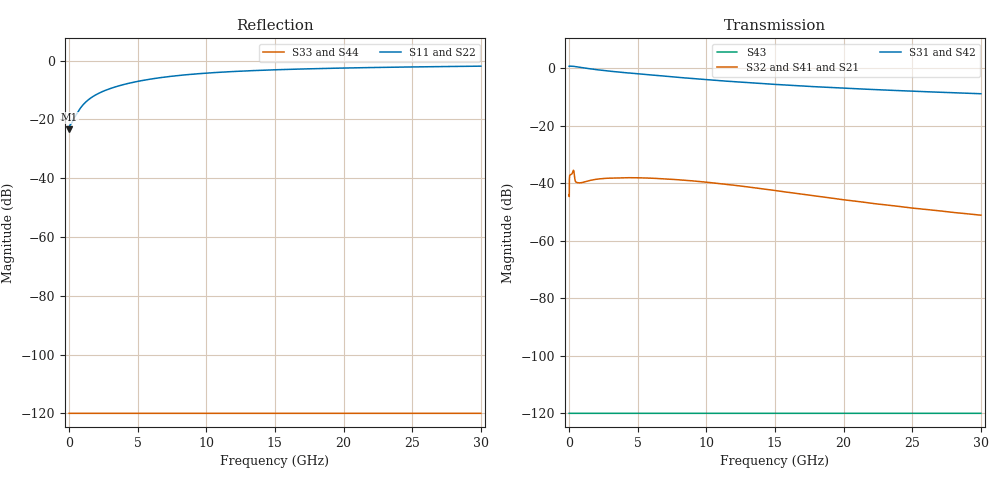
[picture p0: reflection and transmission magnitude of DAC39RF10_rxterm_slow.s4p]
! Copyright 2008, Texas Instruments Incorporated. All rights reserved.
! Generated by program util_convert_RxTerm_to_s4p on 03-29-2011 13:59:15
!  1 ----xxxxxxxxxxxxxxxxxx---- 3
!  xxxxxxxxxxxxxxxxxx
!  (Input) xxxxxxxxxxxxxxxxxx  (Output)
!  xxxxxxxxxxxxxxxxxx
!  2 ----xxxxxxxxxxxxxxxxxx---- 4
! FREQ  S11  S12  S13  S14
!  S21  S22  S23  S24
!  S31  S32  S33  S34
!  S41  S42  S43  S44
!  DB  ANG  DB  ANG  DB  ANG  DB  ANG
# HZ S DB R 50.00
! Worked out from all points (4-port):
!   3000 points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, 10 MHz to 30 GHz, reference 50 ohm
!   strongest paths, dB at 10 MHz, 7.51 GHz, 15.01 GHz, 22.51 GHz, 30 GHz:
!     S31: 0.6, -3.1, -5.7, -7.5, -8.9
!     S42: 0.6, -3.1, -5.7, -7.6, -8.9
!     S32: -44.0, -38.7, -42.6, -47.3, -51.1
!     S41: -44.0, -38.8, -42.7, -47.3, -51.1
!     S21: -44.0, -38.8, -42.7, -47.3, -51.1
!     S43: -120.0, -120.0, -120.0, -120.0, -120.0
!   lowest |S11| = -23.3 dB at 20 MHz (marker M1), VSWR 1.15, Z = 57.3 + j0.0422 ohm
!   |S11| at or under -10 dB: start of sweep to 2.716 GHz
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1e7  -22.90 -3.0  -44.03 -13.4  -120.00 0.0  -120.00 0.0
     -44.00 -13.7  -22.88 -3.0  -120.00 0.0  -120.00 0.0
     0.60 -0.2  -44.03 -13.4  -120.00 0.0  -120.00 0.0
     -44.00 -13.7  0.60 -0.2  -120.00 0.0  -120.00 0.0
2e7  -23.31 0.3  -44.69 58.3  -120.00 0.0  -120.00 0.0
     -44.87 58.3  -23.28 0.3  -120.00 0.0  -120.00 0.0
     0.57 0.0  -44.69 58.3  -120.00 0.0  -120.00 0.0
     -44.87 58.3  0.58 0.0  -120.00 0.0  -120.00 0.0
2.3e8  -20.95 -34.1  -36.63 0.3  -120.00 0.0  -120.00 0.0
       -36.66 0.6  -20.90 -34.2  -120.00 0.0  -120.00 0.0
       0.63 -2.7  -36.63 0.3  -120.00 0.0  -120.00 0.0
       -36.66 0.6  0.63 -2.7  -120.00 0.0  -120.00 0.0
6.4e8  -17.50 -74.0  -39.85 -10.8  -120.00 0.0  -120.00 0.0
       -39.85 -11.0  -17.38 -74.1  -120.00 0.0  -120.00 0.0
       0.38 -7.1  -39.85 -10.8  -120.00 0.0  -120.00 0.0
       -39.85 -11.0  0.38 -7.1  -120.00 0.0  -120.00 0.0
1.9e9  -11.79 -109.7  -38.71 -5.9  -120.00 0.0  -120.00 0.0
       -38.73 -6.1  -11.72 -110.4  -120.00 0.0  -120.00 0.0
       -0.49 -14.9  -38.71 -5.9  -120.00 0.0  -120.00 0.0
       -38.73 -6.1  -0.52 -15.0  -120.00 0.0  -120.00 0.0
6.31e9  -6.02 -134.0  -38.35 -38.8  -120.00 0.0  -120.00 0.0
        -38.46 -39.1  -6.00 -134.2  -120.00 0.0  -120.00 0.0
        -2.56 -28.9  -38.35 -38.8  -120.00 0.0  -120.00 0.0
        -38.46 -39.1  -2.58 -28.9  -120.00 0.0  -120.00 0.0
3e10  -1.89 -160.8  -51.13 -129.0  -120.00 0.0  -120.00 0.0
      -51.10 -128.3  -1.90 -160.9  -120.00 0.0  -120.00 0.0
      -8.93 -47.7  -51.13 -129.0  -120.00 0.0  -120.00 0.0
      -51.10 -128.3  -8.94 -47.5  -120.00 0.0  -120.00 0.0
